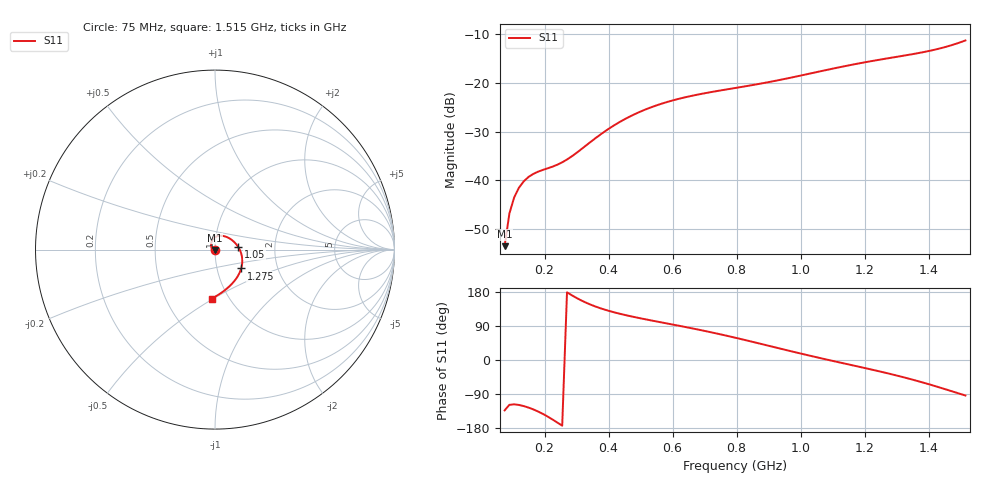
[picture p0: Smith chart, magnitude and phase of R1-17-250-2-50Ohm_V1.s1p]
!version-1
!date-08.2020
!Series
#	GHZ S RI R 50.0
!	FREQ.GHZ	S11RE	S11IM
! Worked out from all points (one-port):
!   97 points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, 75 MHz to 1.515 GHz, reference 50 ohm
!   lowest |S11| = -53.6 dB at 75 MHz (marker M1), VSWR 1.00, Z = 49.9 - j0.153 ohm
!   |S11| at or under -10 dB: start of sweep to end of sweep
!   S11 on the Smith chart (normalised r, x): 75 MHz: 1.00, -0.00; 1.05 GHz: 1.29, +0.04; 1.275 GHz: 1.31, -0.28; 1.515 GHz: 0.83, -0.49
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0.075  -0.00143 -0.00153
0.09  -0.00215 -0.00401
0.105  -0.00302 -0.00594
0.12  -0.00402 -0.00736
0.135  -0.00512 -0.0083
0.15  -0.0063 -0.00878
0.165  -0.00754 -0.00883
0.225  -0.0127 -0.00535
0.255  -0.0152 -0.00176
0.285  -0.0174 0.0028
0.39  -0.0216 0.0237
0.435  -0.0211 0.0337
0.48  -0.0189 0.0435
0.525  -0.0149 0.0528
0.57  -0.00906 0.0611
0.615  -0.00136 0.068
0.69  0.0154 0.0756
0.795  0.0457 0.0759
0.885  0.0757 0.0651
0.975  0.1059 0.0431
1.05  0.1282 0.0163
1.155  0.1489 -0.0334
1.215  0.1519 -0.0674
1.275  0.1459 -0.105
1.335  0.1285 -0.1452
1.425  0.0757 -0.2087
1.47  0.0347 -0.241
1.515  -0.0176 -0.2729
